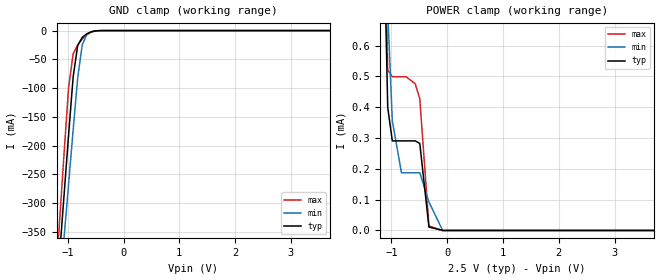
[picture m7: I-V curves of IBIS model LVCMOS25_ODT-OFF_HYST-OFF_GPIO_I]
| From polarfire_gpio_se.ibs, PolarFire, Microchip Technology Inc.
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|   Model LVCMOS25_ODT-OFF_HYST-OFF_GPIO_I
[Model]   LVCMOS25_ODT-OFF_HYST-OFF_GPIO_I
Model_type   Input
Vinl =   0.7
Vinh =   1.7
|   typ   min   max
C_comp_pullup   2.605e-12   2.605e-12   2.76e-12
C_comp_pulldown  2.605e-12   2.605e-12   2.76e-12
[Temperature Range]  25C   100C   -40C
[Voltage Range]  2.5   2.375   2.625
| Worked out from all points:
|   GND clamp passes 1 mA (typ) near -0.52 V on its own axis
|   POWER clamp passes 1 mA (typ) near -1.14 V on its own axis
[GND Clamp]
| Voltage   I(typ)   I(min)   I(max)
-2.5V     -2.154A    -2.019A    -2.334A
-1.312V   -606.5mA   -644.5mA   -576.7mA
-1.148V   -394.1mA   -456mA     -335.8mA
-1.066V   -288mA     -361.7mA   -215.7mA
-984.4mV  -181.9mA   -267.4mA   -99.94mA
-902.3mV  -80.78mA   -173.2mA   -40.34mA
-820.3mV  -25.8mA    -81.78mA   -25.07mA
-738.3mV  -11.65mA   -24.31mA   -14.68mA
-656.2mV  -5.525mA   -6.674mA   -7.068mA
-574.2mV  -1.954mA   -1.999mA   -2.52mA
-410.2mV  -41.8uA    -66.55uA   -50.18uA
5V        0A         0A         0A
[POWER Clamp]
| Voltage   I(typ)   I(min)   I(max)
-2.5V     56.69mA    37.57mA    83.75mA
-1.148V   1.079mA    1.117mA    1.211mA
-1.066V   399uA      709.9uA    520.5uA
-984.4mV  290.7uA    355.8uA    498.9uA
-820.3mV  290.7uA    187.2uA    498.9uA
-738.3mV  290.7uA    187.2uA    498.9uA
-574.2mV  290.7uA    187.2uA    475.9uA
-492.2mV  282.4uA    187.2uA    427.6uA
-328.1mV  11.03uA    92.62uA    14.81uA
-82.03mV  104.8nA    31.48nA    2.661nA
5V        0A         0A         0A
